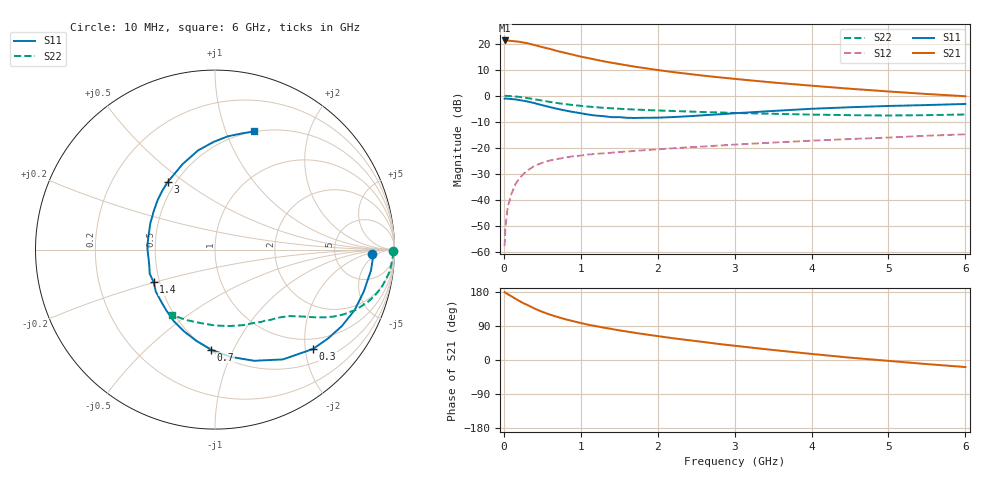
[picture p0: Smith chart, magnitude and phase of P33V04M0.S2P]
! SIEMENS Small Signal Semiconductors
! BFP181
! Si NPN RF Bipolar Junction Transistor in SOT143
! VCE = 3 V  IC = 4 mA
! Common Emitter S-Parameters:  March  1996
# GHz  S  MA  R  50
!  f  S11  S21  S12  S22
! GHz  MAG  ANG  MAG  ANG  MAG  ANG  MAG  ANG
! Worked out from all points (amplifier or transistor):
!   36 points, 10 MHz to 6 GHz, reference 50 ohm
!   highest |S21| = 21.2 dB at 10 MHz (marker M1)
!   |S21| within 3 dB of that: start of sweep to 563.1 MHz
!   unconditionally stable (mu >= 1): 1.863 GHz to end of sweep
!   at 250 MHz: K = 0.19, MSG = 25.3 dB, |S12| = -30.2 dB
!   at 1.4 GHz: K = 0.85, MSG = 17.3 dB, |S12| = -21.9 dB
!   at 6 GHz: K = 1.07, MAG = 5.7 dB, |S12| = -14.8 dB
!   S11 on the Smith chart (normalised r, x): 10 MHz: 14, -3; 300 MHz: 0.77, -2.16; 700 MHz: 0.51, -0.82; 1.4 GHz: 0.46, -0.20; 3 GHz: 0.45, +0.43; 6 GHz: 0.50, +1.26
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0.01  0.8746 -1.7  11.46 178.8  0.0013 77.7  0.9928 -0.6
0.02  0.8809 -3.2  11.45 177.9  0.0029 85.5  0.9931 -1.4
0.05  0.8768 -7.6  11.39 173.8  0.0073 86.8  0.989 -3.5
0.1  0.8611 -15.8  11.21 167.9  0.0132 79.3  0.9822 -6.8
0.2  0.8252 -31.1  10.81 156.0  0.0257 72.6  0.9484 -13.2
0.25  0.801 -38.2  10.47 150.4  0.0309 69.1  0.926 -16.1
0.3  0.7776 -45.4  10.17 145.7  0.0363 66.1  0.9022 -18.7
0.4  0.7192 -58.3  9.364 135.6  0.0451 60.3  0.8538 -23.1
0.5  0.6563 -70.7  8.533 127.1  0.0517 54.3  0.8043 -26.6
0.6  0.6034 -81.9  7.873 119.8  0.0573 50.4  0.7596 -29.4
0.7  0.5578 -92.2  7.151 113.4  0.0612 47.4  0.7202 -31.6
0.8  0.5187 -101.6  6.613 107.6  0.0651 45.0  0.6877 -33.3
0.9  0.4871 -110.7  6.09 102.5  0.0688 42.8  0.6614 -34.7
1.1  0.4335 -128.9  5.249 93.0  0.0744 39.9  0.6166 -37.2
1.4  0.387 -152.2  4.285 81.9  0.0806 37.2  0.5727 -40.4
1.8  0.3763 -180.0  3.429 68.8  0.0896 35.5  0.5345 -44.5
2.2  0.3892 157.8  2.833 57.4  0.0981 33.6  0.5082 -49.3
3  0.46 124.9  2.1 37.6  0.1151 30.7  0.4658 -60.8
3.5  0.5093 110.8  1.788 26.4  0.1262 28.3  0.4495 -69.4
4.5  0.6002 90.7  1.359 6.2  0.1473 22.8  0.4231 -89.8
5.5  0.6611 77.6  1.077 -10.8  0.1703 18.0  0.4233 -111.8
6  0.6936 71.8  0.975 -18.6  0.182 14.4  0.4354 -123.1
